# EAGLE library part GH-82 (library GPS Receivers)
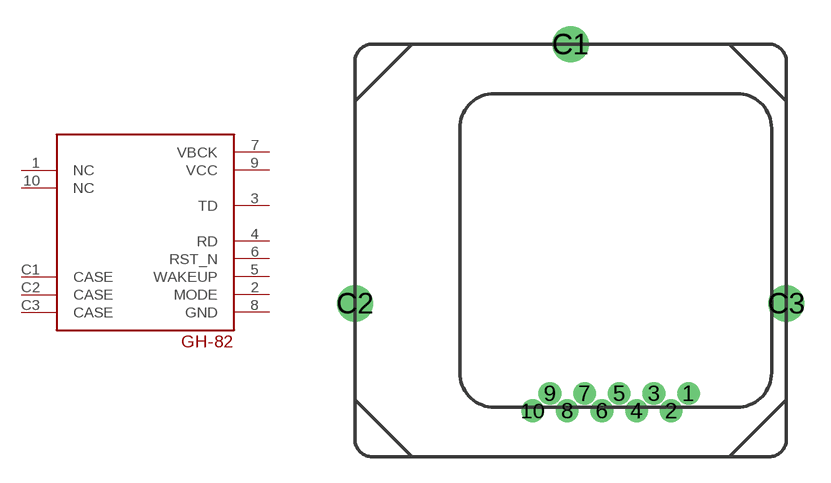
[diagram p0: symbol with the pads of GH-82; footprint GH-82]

Designator prefix U

## GH-82  [GH-82]
1  NC  nc
2  MODE
3  TD  out
4  RD  in
5  WAKEUP  in
6  RST_N  in
7  VBCK  in
8  GND
9  VCC
10  NC  nc
C1  CASE
C2  CASE
C3  CASE

## Footprint GH-82 (pad centres in mm)
drill 0.8 pad 1: 1 6.8,-5.2; 2 5.8,-6.2; 3 4.8,-5.2; 4 3.8,-6.2; 5 2.8,-5.2; 6 1.8,-6.2; 7 0.8,-5.2; 8 -0.2,-6.2; 9 -1.2,-5.2; 10 -2.2,-6.2
drill 1.4: C1 0,14.95; C2 -12.45,0; C3 12.45,0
